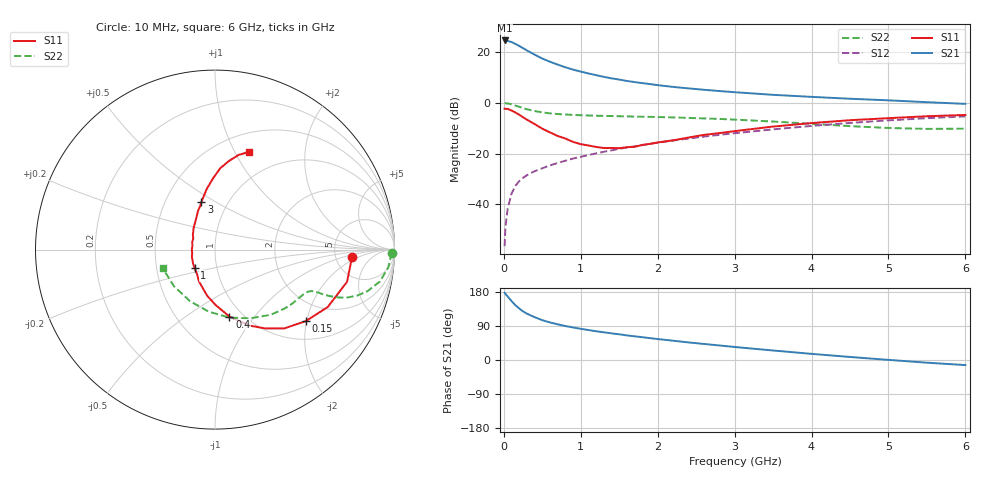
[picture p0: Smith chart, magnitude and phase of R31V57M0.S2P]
! SIEMENS Small Signal Semiconductors
! BFR181
! Si NPN RF Bipolar Junction Transistor in SOT23
! VCE = 1.5 V  IC = 7 mA
! Common Emitter S-Parameters:  May  1996
# GHz  S  MA  R  50
!  f  S11  S21  S12  S22
! GHz  MAG  ANG  MAG  ANG  MAG  ANG  MAG  ANG
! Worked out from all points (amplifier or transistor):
!   36 points, 10 MHz to 6 GHz, reference 50 ohm
!   highest |S21| = 24.6 dB at 10 MHz (marker M1)
!   |S21| within 3 dB of that: start of sweep to 247 MHz
!   unconditionally stable (mu >= 1): 808.8 MHz to 2.849 GHz
!   at 250 MHz: K = 0.54, MSG = 25.5 dB, |S12| = -29.6 dB
!   at 1.4 GHz: K = 1.09, MAG = 12.4 dB, |S12| = -18.7 dB
!   at 6 GHz: K = 0.87, MSG = 2.5 dB, |S12| = -5.4 dB
!   S11 on the Smith chart (normalised r, x): 10 MHz: 7.29, -1.42; 150 MHz: 1.45, -1.98; 400 MHz: 0.87, -0.76; 1 GHz: 0.78, -0.16; 3 GHz: 0.75, +0.43; 6 GHz: 0.70, +1.14
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0.01  0.7668 -3.0  16.92 177.5  0.0015 86.3  0.9847 -1.1
0.02  0.7602 -5.8  16.7 174.7  0.0035 86.1  0.9803 -2.4
0.05  0.7573 -13.7  16.54 167.4  0.0082 83.4  0.9704 -5.9
0.1  0.7049 -27.0  15.76 155.6  0.0163 78.3  0.9351 -11.0
0.15  0.6441 -38.2  14.43 144.6  0.0231 71.5  0.8814 -15.2
0.2  0.584 -48.8  13.19 136.0  0.0287 69.1  0.8329 -17.9
0.25  0.519 -57.7  11.91 128.3  0.0333 66.2  0.7865 -19.8
0.3  0.466 -65.4  10.74 122.2  0.0375 65.9  0.7458 -21.0
0.4  0.3819 -77.8  8.893 113.1  0.0449 64.5  0.6886 -22.1
0.5  0.3091 -89.3  7.444 105.1  0.0514 64.2  0.6482 -22.5
0.6  0.2611 -99.6  6.436 99.1  0.0586 64.7  0.6195 -22.6
0.8  0.198 -116.8  5.013 89.7  0.0724 65.4  0.5885 -23.1
1  0.1533 -138.0  4.115 82.3  0.0864 66.3  0.5695 -24.3
1.1  0.1444 -148.1  3.789 79.1  0.0937 66.8  0.563 -25.0
1.3  0.1289 -170.4  3.242 73.1  0.1086 66.9  0.5522 -26.7
1.6  0.1336 162.1  2.696 64.9  0.1314 66.4  0.5402 -29.8
2.2  0.1823 128.5  2.059 50.9  0.1808 64.1  0.5156 -38.0
3  0.2769 105.8  1.618 34.4  0.2518 58.4  0.4668 -51.9
3.5  0.3407 97.8  1.437 25.1  0.3001 54.0  0.4282 -63.6
4.5  0.4544 86.3  1.203 8.0  0.4016 42.7  0.3471 -96.0
5.5  0.544 76.0  1.029 -7.1  0.498 29.4  0.3065 -138.3
6  0.5768 70.7  0.954 -13.4  0.54 22.2  0.3095 -160.6
